(* Logix 5000 AddOnInstructionDefinition export; software revision 16.04 *)

ADD_ON_INSTRUCTION AMCI_ANG1E_Jog_CCW   (* revision 1.1, vendor AMCI, ExecuteEnableInFalse *)
// Revision note:
// Version 1.1 added the slot_axis number and the input parameters can now be tags or discrete values.
VAR_INPUT
   Axis_Status_Bits : DINT; {required}
   slot_axis_number : INT; {required}
   Programmed_Speed : DINT; {required}
   Acceleration : INT; {required}
   Deceleration : INT; {required}
   jerk : INT;
END_VAR
VAR_IN_OUT
   AMCI_ANG1E_output_data : INT[10]; {required}
END_VAR
VAR_OUTPUT
   EN : BOOL; {visible}
   Jog_CCW_Occurring : BOOL; {visible}
   ER : BOOL; {visible}
END_VAR
VAR
   Upper_Result_X_1000 : DINT;
   command_data_block : INT[10];
        [0]   // Command Bits MSW
        [1]   // Command Bits LSW
        [2]   // Upper Target Position
        [3]   // Lower Target Position
        [4]   // Upper Programmed Speed
        [5]   // Lower Programmed Speed
   index : INT;
END_VAR

ROUTINE EnableInFalse   (* ladder *)
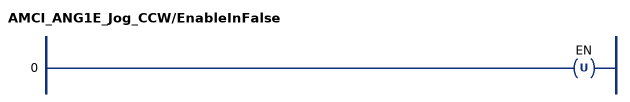
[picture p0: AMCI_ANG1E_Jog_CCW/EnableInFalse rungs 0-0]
   0: OTU(EN);
END_ROUTINE

ROUTINE Logic   (* ladder *)
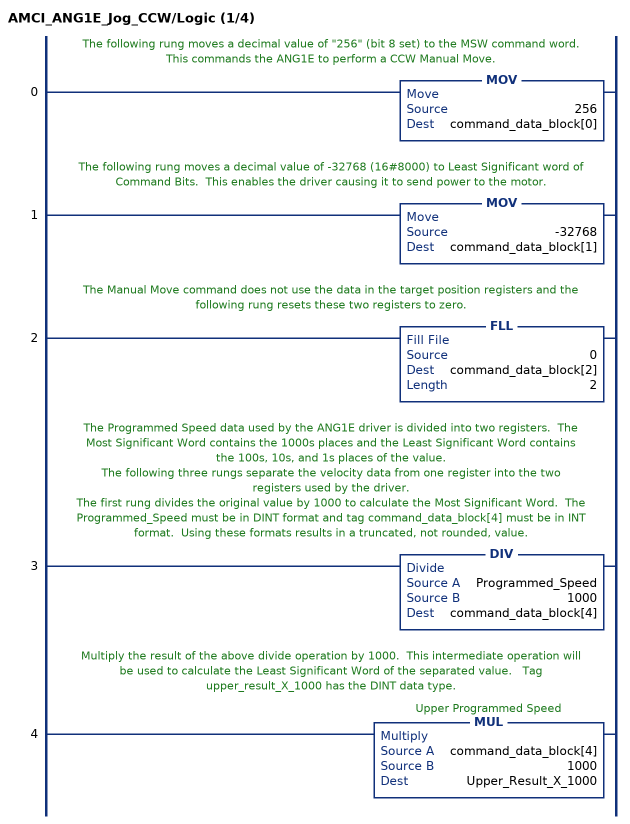
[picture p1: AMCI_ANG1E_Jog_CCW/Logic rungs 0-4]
   // The following rung moves a decimal value of "256" (bit 8 set) to the MSW command word.  This commands the ANG1E to perform a CCW Manual Move.
   0: MOV(256,command_data_block[0]);
   // The following rung moves a decimal value of -32768 (16#8000) to Least Significant word of Command Bits.  This enables the driver causing it to send power to the motor.
   1: MOV(-32768,command_data_block[1]);
   // The Manual Move command does not use the data in the target position registers and the following rung resets these two registers to zero.
   2: FLL(0,command_data_block[2],2);
   // The Programmed Speed data used by the ANG1E driver is divided into two registers.  The Most Significant Word contains the 1000s places and the Least Significant Word contains the 100s, 10s, and 1s places of the value.
   // The following three rungs separate the velocity data from one register into the two registers used by the driver.
   // The first rung divides the original value by 1000 to calculate the Most Significant Word.  The Programmed_Speed must be in DINT format and tag command_data_block[4] must be in INT format.  Using these formats results in a truncated, not rounded, value.
   3: DIV(Programmed_Speed,1000,command_data_block[4]);
   // Multiply the result of the above divide operation by 1000.  This intermediate operation will be used to calculate the Least Significant Word of the separated value.   Tag upper_result_X_1000 has the DINT data type.
   4: MUL(command_data_block[4],1000,Upper_Result_X_1000);
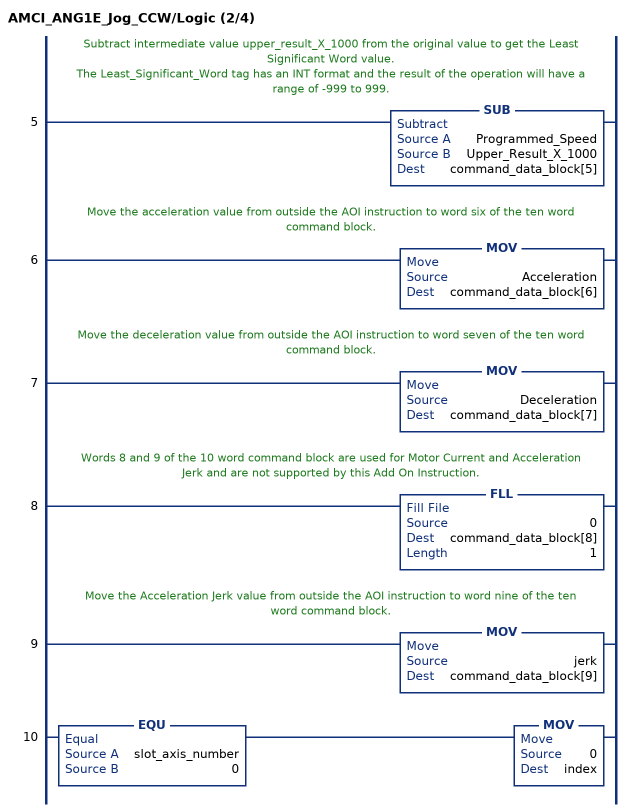
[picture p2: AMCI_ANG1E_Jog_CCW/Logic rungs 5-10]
   // Subtract intermediate value upper_result_X_1000 from the original value to get the Least Significant Word value.
   // The Least_Significant_Word tag has an INT format and the result of the operation will have a range of -999 to 999.
   5: SUB(Programmed_Speed,Upper_Result_X_1000,command_data_block[5]);
   // Move the acceleration value from outside the AOI instruction to word six of the ten word command block.
   6: MOV(Acceleration,command_data_block[6]);
   // Move the deceleration value from outside the AOI instruction to word seven of the ten word command block.
   7: MOV(Deceleration,command_data_block[7]);
   // Words 8 and 9 of the 10 word command block are used for Motor Current and Acceleration Jerk and are not supported by this Add On Instruction.
   8: FLL(0,command_data_block[8],1);
   // Move the Acceleration Jerk value from outside the AOI instruction to word nine of the ten word command block.
   9: MOV(jerk,command_data_block[9]);
   10: EQU(slot_axis_number,0)MOV(0,index);
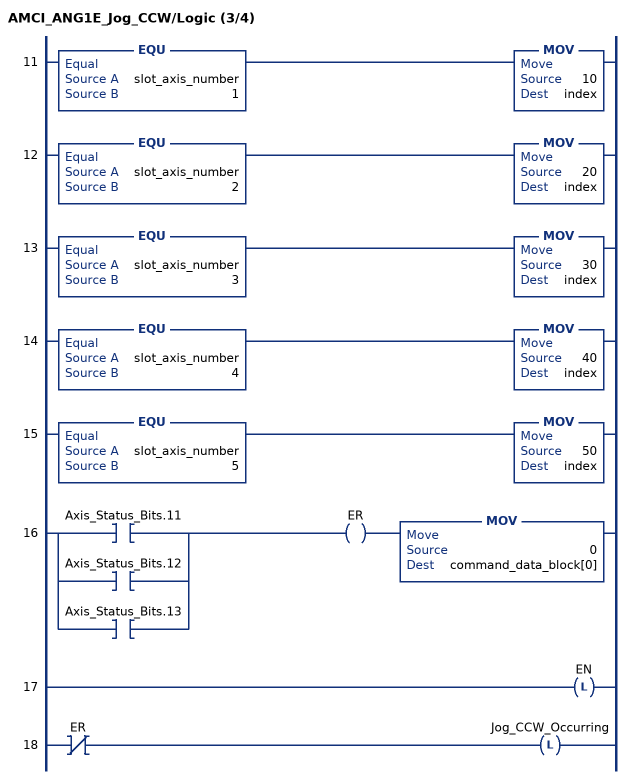
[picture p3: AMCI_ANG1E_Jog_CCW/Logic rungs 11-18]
   11: EQU(slot_axis_number,1)MOV(10,index);
   12: EQU(slot_axis_number,2)MOV(20,index);
   13: EQU(slot_axis_number,3)MOV(30,index);
   14: EQU(slot_axis_number,4)MOV(40,index);
   15: EQU(slot_axis_number,5)MOV(50,index);
   16: [XIC(Axis_Status_Bits.11) ,XIC(Axis_Status_Bits.12) ,XIC(Axis_Status_Bits.13) ]OTE(ER)MOV(0,command_data_block[0]);
   17: OTL(EN);
   18: XIO(ER)OTL(Jog_CCW_Occurring);
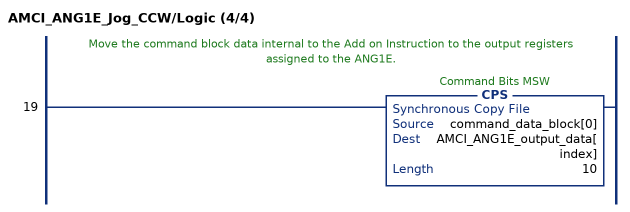
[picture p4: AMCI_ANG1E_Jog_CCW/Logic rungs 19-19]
   // Move the command block data internal to the Add on Instruction to the output registers assigned to the ANG1E.
   19: CPS(command_data_block[0],AMCI_ANG1E_output_data[index],10);
END_ROUTINE
END_ADD_ON_INSTRUCTION
